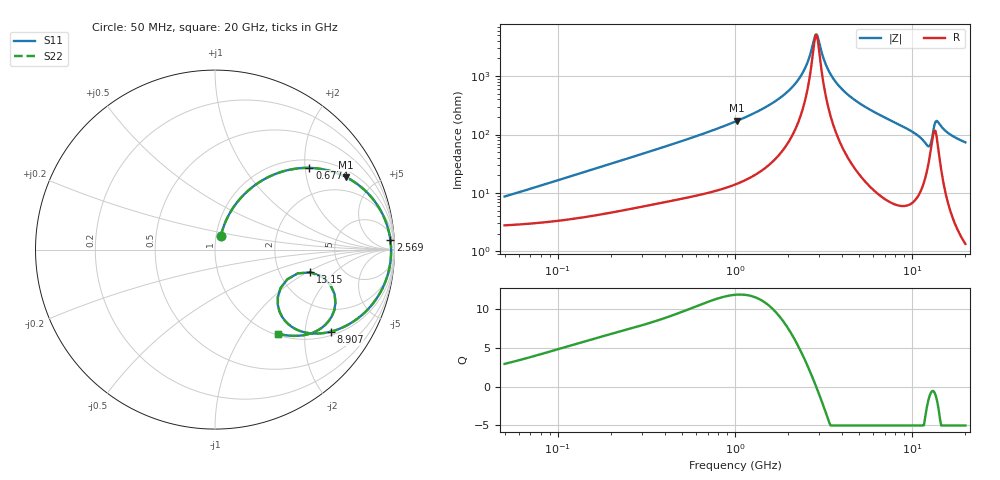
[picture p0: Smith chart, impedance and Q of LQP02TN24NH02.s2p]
!Murata Part Number: LQP02TN24NH02
!These Parameters are Measured in Series Mode Connection
!  o--[Z]--o
!Port1  Port2
!  o-------o
!Freq. Start=50[MHz] Stop=20[GHz], 401[Steps]
# Hz S RI R 50
!Freq.(Hz) S11(Real) S11(Imag) S21(Real) S21(Imag) S12(Real) S12(Imag) S22(Real) S22(Imag)
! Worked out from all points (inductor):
!   401 points, 50 MHz to 20 GHz, reference 50 ohm
!   read as one part in series: L = 26 nH near 51.52 MHz
!   highest Q = 11.9 at 1.03 GHz (marker M1), where L = 26.5 nH
!   self-resonance near 2.853 GHz
!   S11 on the Smith chart (normalised r, x): 50 MHz: 1.06, +0.16; 677.4 MHz: 1.19, +2.11; 2.569 GHz: 13, +32; 8.907 GHz: 1.12, -2.72; 13.15 GHz: 2.98, -1.08; 20 GHz: 1.03, -1.47
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5e7  0.0333 0.0774  0.9667 -0.0774  0.9667 -0.0774  0.0333 0.0774
1.364002e8  0.0771 0.1936  0.9229 -0.1936  0.9229 -0.1936  0.0771 0.1936
3.721004e8  0.2714 0.3904  0.7286 -0.3904  0.7286 -0.3904  0.2714 0.3904
6.774326e8  0.5255 0.4553  0.4745 -0.4553  0.4745 -0.4553  0.5255 0.4553
1e9  0.7167 0.4104  0.2833 -0.4104  0.2833 -0.4104  0.7167 0.4104
1.030411e9  0.7306 0.4036  0.2694 -0.4036  0.2694 -0.4036  0.7306 0.4036
1.875929e9  0.9355 0.1933  0.0645 -0.1933  0.0645 -0.1933  0.9355 0.1933
2.279204e9  0.9669 0.107  0.0331 -0.107  0.0331 -0.107  0.9669 0.107
2.569357e9  0.9774 0.0521  0.0226 -0.0521  0.0226 -0.0521  0.9774 0.0521
2.728004e9  0.9802 0.0243  0.0198 -0.0243  0.0198 -0.0243  0.9802 0.0243
2.810964e9  0.981 0.0104  0.019 -0.0104  0.019 -0.0104  0.981 0.0104
2.896447e9  0.9813 -0.00362  0.0187 0.00362  0.0187 0.00362  0.9813 -0.00362
3.364474e9  0.9767 -0.0737  0.0233 0.0737  0.0233 0.0737  0.9767 -0.0737
4.149438e9  0.952 -0.1716  0.048 0.1716  0.048 0.1716  0.952 -0.1716
7.442007e9  0.7529 -0.4121  0.2471 0.4121  0.2471 0.4121  0.7529 -0.4121
8.907419e9  0.6437 -0.4575  0.3563 0.4575  0.3563 0.4575  0.6437 -0.4575
1.098561e10  0.4615 -0.4486  0.5385 0.4486  0.5385 0.4486  0.4615 -0.4486
1.220001e10  0.35 -0.308  0.65 0.308  0.65 0.308  0.35 -0.308
1.314879e10  0.5313 -0.1267  0.4687 0.1267  0.4687 0.1267  0.5313 -0.1267
1.396067e10  0.6713 -0.2976  0.3287 0.2976  0.3287 0.2976  0.6713 -0.2976
1.527346e10  0.5775 -0.447  0.4225 0.447  0.4225 0.447  0.5775 -0.447
2e10  0.3525 -0.4687  0.6475 0.4687  0.6475 0.4687  0.3525 -0.4687
